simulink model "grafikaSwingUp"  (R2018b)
settings: Solver=ode4  StartTime=0.0  StopTime=1.85  FixedStep=1e-3  RelTol=1e-3
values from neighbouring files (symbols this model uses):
  dtheta0 = [dtheta0 , stbVc]    [mainSkript_provedeniSimulaceSwingUp.m]    (also in mainSkript_odhadKyvadlaZvlast.m = mean(dtheta(n_start-5:n_start+5)); mainSkript_pocitaniTVLQR_simplified.m = traj.dth_0)
  dtheta1 = [dtheta1 , stbVc]    [mainSkript_provedeniSimulaceSwingUp.m]    (also in mainSkript_pocitaniTVLQR_simplified.m = traj.dth_1)
  dtheta2 = [dtheta2 , stbVc]    [mainSkript_provedeniSimulaceSwingUp.m]    (also in mainSkript_pocitaniTVLQR_simplified.m = traj.dth_2)
  g = 9.81    [mainSkript_provedeniSimulaceSwingUp.m]    (also in mainSkript_rovniceSystemu.m; mainSkript_overeniRovnic.m; mainSkript_estimaceVozik.m; mainSkript_odhadKyvadlaZvlast.m)
  I_1 = params.I_1    [mainSkript_provedeniSimulaceSwingUp.m]    (also in mainSkript_rovniceSystemu.m; mainSkript_overeniRovnic.m; mainSkript_kyvadlaNajednouOdhad.m; mainSkript_simulaceLQG.m)
  I_2 = params.I_2    [mainSkript_provedeniSimulaceSwingUp.m]    (also in mainSkript_rovniceSystemu.m; mainSkript_overeniRovnic.m; mainSkript_kyvadlaNajednouOdhad.m; mainSkript_simulaceLQG.m)
  l_1 = params.l_1    [mainSkript_provedeniSimulaceSwingUp.m]    (also in mainSkript_rovniceSystemu.m; mainSkript_overeniRovnic.m; odhadovane_parametry.m = 0.134; mainSkript_kyvadlaNajednouOdhad.m)
  L_1 = params.L_1    [mainSkript_provedeniSimulaceSwingUp.m]    (also in mainSkript_rovniceSystemu.m; mainSkript_overeniRovnic.m; odhadovane_parametry.m = 0.228; mainSkript_kyvadlaNajednouOdhad.m)
  l_2 = params.l_2    [mainSkript_provedeniSimulaceSwingUp.m]    (also in mainSkript_rovniceSystemu.m; mainSkript_overeniRovnic.m; odhadovane_parametry.m = 0.112; mainSkript_kyvadlaNajednouOdhad.m)
  m = params.m_0    [mainSkript_estimaceVozik.m]    (also in mainSkript_odhadKyvadlaZvlast.m = params.m_2; mainSkript_modifikaceVozik.m = 1.437)
  m_0 = params.m_0    [mainSkript_provedeniSimulaceSwingUp.m]    (also in mainSkript_rovniceSystemu.m; mainSkript_overeniRovnic.m; mainSkript_simulaceLQG.m; mainSkript_LQGexperiment.m)
  m_1 = params.m_1    [mainSkript_provedeniSimulaceSwingUp.m]    (also in mainSkript_rovniceSystemu.m; mainSkript_overeniRovnic.m; mainSkript_kyvadlaNajednouOdhad.m; mainSkript_simulaceLQG.m)
  m_2 = params.m_2    [mainSkript_provedeniSimulaceSwingUp.m]    (also in mainSkript_rovniceSystemu.m; mainSkript_overeniRovnic.m; mainSkript_kyvadlaNajednouOdhad.m; mainSkript_simulaceLQG.m)
  N = N * Cref'    [mainSkript_simulaceLQG.m]    (also in mainSkript_tvorbaTrajektorii.m = 100; mainSkript_pocitaniTVLQR_simplified.m = floor( length(time) / krok ))
  theta0 = [theta0 , stbVc]    [mainSkript_provedeniSimulaceSwingUp.m]    (also in mainSkript_odhadKyvadlaZvlast.m = theta_cut(1); mainSkript_pocitaniTVLQR_simplified.m = traj.th_0)
  theta1 = [theta1 , stbVc]    [mainSkript_provedeniSimulaceSwingUp.m]    (also in mainSkript_kyvadlaNajednouOdhad.m = pend.theta1; mainSkript_pocitaniTVLQR_simplified.m = traj.th_1)
  theta2 = [theta2 , stbVc]    [mainSkript_provedeniSimulaceSwingUp.m]    (also in mainSkript_kyvadlaNajednouOdhad.m = pend.theta2; mainSkript_pocitaniTVLQR_simplified.m = traj.th_2)
undefined symbols (not defined in the file or in its folder): DiscIntNeverNeededParam, kg, rad, s
libraries: mblibv1 x14

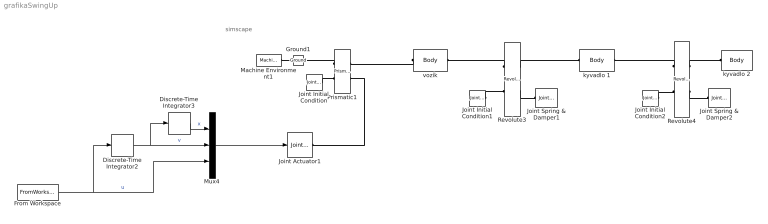
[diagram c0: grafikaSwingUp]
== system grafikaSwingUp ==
  note: simscape
  Discrete-Time Integrator2 : DiscreteIntegrator  SampleTime=1e-3  ICPrevOutput=DiscIntNeverNeededParam  ICPrevScaledInput=DiscIntNeverNeededParam
  Discrete-Time Integrator3 : DiscreteIntegrator  SampleTime=1e-3  ICPrevOutput=DiscIntNeverNeededParam  ICPrevScaledInput=DiscIntNeverNeededParam
  From Workspace : FromWorkspace  VariableName=u_str  SampleTime=0
  Ground1 : mblibv1/Bodies/Ground  UpdateFromCAD=off  LeftPortType=env  RightPortType=workingframe  PhysicalDomain=Mechanical  DialogClass=GroundBlock  CoordPosition=[0 0 0]  CoordPositionUnits=m  StateVectorMgrId=0  MachineId=[1 0]  ShowEnvPort=on  ParameterChecksum=[1834074738, 1660941931, 768696267, 1500060636]  TopologyChecksum=[1367285865, 302751694, 2522931292, 506890735]
  Joint Actuator1 : mblibv1/Sensors &  Actuators/Joint Actuator  UpdateFromCAD=off  PhysicalDomain=Mechanical  PortType=blob  ActuationStyle=Motion  AngleUnits=rad  ArcVelocityUnits=rad/s  ArcAccelerationUnits=rad/s^2  CoordPositionUnits=m  VelocityUnits=m/s  AccelerationUnits=m/s^2  ForceUnits=N  TorqueUnits=N*m  ActiveIO=on  Width=3  DialogClass=MechanicalActuatorBlock  Primitive=P1  ReferenceFrame=Absolute (World)
  Joint Initial Condition : mblibv1/Sensors &  Actuators/Joint Initial Condition  UpdateFromCAD=off  LeftPortType=blob  RightPortType=blob  PhysicalDomain=mechanical  DialogClass=InitialConditionBlock  InitialConditions=P1$true$theta0(1)$m$deg$dtheta0(1)$m/s$deg/s#P2$false$0$m$deg$0$m/s$deg/s#P3$false$0$m$deg$0$m/s$deg/s#R1$false$0$m$deg$0$m/s$deg/s#R2$false$0$m$deg$0$m/s$deg/s#R3$false$0$m$deg$0$m/s$deg/s#S$false$0$m$deg$0$m/s$deg/s  P1PIC=theta0(1)  P1VIC=dtheta0(1)  P2PIC=0  P2VIC=0  P3PIC=0  P3VIC=0  R1PIC=0  R1VIC=0  R2PIC=0  R2VIC=0  R3PIC=0  R3VIC=0  SPIC=0  SVIC=0
  Joint Initial Condition1 : mblibv1/Sensors &  Actuators/Joint Initial Condition  UpdateFromCAD=off  LeftPortType=blob  RightPortType=blob  PhysicalDomain=mechanical  DialogClass=InitialConditionBlock  InitialConditions=P1$false$th0i$m$deg$dth0i$m/s$deg/s#P2$false$0$m$deg$0$m/s$deg/s#P3$false$0$m$deg$0$m/s$deg/s#R1$true$theta1(1)$m$rad$dtheta1(1)$m/s$rad/s#R2$false$0$m$deg$0$m/s$deg/s#R3$false$0$m$deg$0$m/s$deg/s#S$false$0$m$deg$0$m/s$deg/s  P1PIC=0  P1VIC=0  P2PIC=0  P2VIC=0  P3PIC=0  P3VIC=0  R1PIC=theta1(1)  R1VIC=dtheta1(1)  R2PIC=0  R2VIC=0  R3PIC=0  R3VIC=0  SPIC=0  SVIC=0
  Joint Initial Condition2 : mblibv1/Sensors &  Actuators/Joint Initial Condition  UpdateFromCAD=off  LeftPortType=blob  RightPortType=blob  PhysicalDomain=mechanical  DialogClass=InitialConditionBlock  InitialConditions=P1$false$th0i$m$deg$dth0i$m/s$deg/s#P2$false$0$m$deg$0$m/s$deg/s#P3$false$0$m$deg$0$m/s$deg/s#R1$true$theta2(1) - theta1(1)$m$rad$dtheta2(1) - dtheta1(1)$m/s$rad/s#R2$false$0$m$deg$0$m/s$deg/s#R3$false$0$m$deg$0$m/s$deg/s#S$false$0$m$deg$0$m/s$deg/s  P1PIC=0  P1VIC=0  P2PIC=0  P2VIC=0  P3PIC=0  P3VIC=0  R1PIC=theta2(1) - theta1(1)  R1VIC=dtheta2(1) - dtheta1(1)  R2PIC=0  R2VIC=0  R3PIC=0  R3VIC=0  SPIC=0  SVIC=0
  Joint Spring & Damper1 : mblibv1/Force  Elements/Joint Spring & Damper  UpdateFromCAD=off  DialogClass=JointSpringDamper  JFEParameters=P1$false$0$b0$0$m$m/s$N$deg$deg/s$N*m#P2$false$0$0$0$m$m/s$N$deg$deg/s$N*m#P3$false$0$0$0$m$m/s$N$deg$deg/s$N*m#R1$true$0$b_1$0$m$m/s$N$rad$rad/s$N*m#R2$false$0$0$0$m$m/s$N$deg$deg/s$N*m#R3$false$0$0$0$m$m/s$N$deg$deg/s$N*m#S$false$0$0$0$m$m/s$N$deg$deg/s$N*m
  Joint Spring & Damper2 : mblibv1/Force  Elements/Joint Spring & Damper  UpdateFromCAD=off  DialogClass=JointSpringDamper  JFEParameters=P1$false$0$b0$0$m$m/s$N$deg$deg/s$N*m#P2$false$0$0$0$m$m/s$N$deg$deg/s$N*m#P3$false$0$0$0$m$m/s$N$deg$deg/s$N*m#R1$true$0$b_2$0$m$m/s$N$rad$rad/s$N*m#R2$false$0$0$0$m$m/s$N$deg$deg/s$N*m#R3$false$0$0$0$m$m/s$N$deg$deg/s$N*m#S$false$0$0$0$m$m/s$N$deg$deg/s$N*m
  Machine Environment1 : mblibv1/Bodies/Machine Environment  PortType=env  PhysicalDomain=Mechanical  DialogTemplateClass=MECH.MachineEnvironment  SyncWhenCopied=off  Gravity=[0 -g 0]  GravityUnits=m/s^2  GravityAsSignal=off  Dimensionality=Auto-detect  AnalysisType=Forward dynamics  LinearAssemblyTolerance=1e-3  LinearAssemblyToleranceUnits=m  AngularAssemblyTolerance=1e-3  AngularAssemblyToleranceUnits=rad  ConstraintSolverType=Stabilizing  ConstraintRelTolerance=1e-4  ConstraintAbsTolerance=1e-4  UseRobustSingularityHandling=off  RedundancyAnalysisToleranceType=Automatically select tolerance  RedundancyAnalysisTolerance=1e-14  StatePerturbationType=Fixed  PerturbationSize=1e-5  VisualizeMachine=on  BodyVisualizationType=Use model default body geometries  BodyColorSelMode=Use model default  DefaultBodyColor=[1 0 0]
  Mux4 : Mux  Inputs=3
  Prismatic1 : mblibv1/Joints/Prismatic  LConnTagsString=__newl0|SA1  RConnTagsString=__newr0|SA1  UpdateFromCAD=off  NumSAPorts=2  CutJoint=off  MarkAsCut=off  Primitives=prismatic  PrimitiveProps=P1$World$[-1 0 0]$prismatic  DialogClass=JointBlock  P1Axis=[-1 0 0]
  Revolute3 : mblibv1/Joints/Revolute  LConnTagsString=__newl0|SA1  RConnTagsString=__newr0|SA1  UpdateFromCAD=off  NumSAPorts=2  CutJoint=off  MarkAsCut=off  Primitives=prismatic  PrimitiveProps=R1$World$[0 0 1]$revolute  DialogClass=JointBlock  R1Axis=[0 0 1]
  Revolute4 : mblibv1/Joints/Revolute  LConnTagsString=__newl0|SA1  RConnTagsString=__newr0|SA1  UpdateFromCAD=off  NumSAPorts=2  CutJoint=off  MarkAsCut=off  Primitives=prismatic  PrimitiveProps=R1$Base$[0 0 1]$revolute  DialogClass=JointBlock  R1Axis=[0 0 1]
  kyvadlo 1 : mblibv1/Bodies/Body  LConnTagsString=CS1  RConnTagsString=CS2  UpdateFromCAD=off  DialogClass=MechanicalBodyBlock  Mass=m_1  MassUnits=kg  InertiaUnits=kg*m^2  Inertia=eye(3)*I_1  Shape=Cylinder  ShapeDims=[1 1]  ShapeUnits=m  ShapeUse=false  Density=1  DensityUnits=kg/m^3  DensityUse=false  GraphicsMode=MACHINE_DEFAULT  BodyColorSelMode=COLORPALETTE  BodyColor=[0 0 0]  AttachedToCS=CG  CG=Left$CG$[0 l_1 0]$CS1$CS1$m$[0 0 0]$Euler X-Y-Z$deg$WORLD$false$none  WorkingFrames=Left$CS1$[0 0 0]$Adjoining$Adjoining$m$[0 0 0]$Euler X-Y-Z$deg$WORLD$true$none#Right$CS2$[0 L_1 0]$CS1$CS1$m$[0 0 0]$Euler X-Y-Z$deg$WORLD$true$none  CGPos=[0 l_1 0]  CGRot=[0 0 0]  CS0Pos=[]  CS0Rot=[]  CS1Pos=[0 0 0]  CS1Rot=[0 0 0]  CS2Pos=[0 L_1 0]  CS2Rot=[0 0 0]  CS3Pos=[]  CS3Rot=[]  CS4Pos=[]  CS4Rot=[]  CS5Pos=[]  CS5Rot=[]  CS6Pos=[]  CS6Rot=[]  CS7Pos=[]  CS7Rot=[]  CS8Pos=[]  CS8Rot=[]  CS9Pos=[]  CS9Rot=[]  CS10Pos=[]  CS10Rot=[]  CS11Pos=[]  CS11Rot=[]  CS12Pos=[]  CS12Rot=[]  CS13Pos=[]  CS13Rot=[]  CS14Pos=[]  CS14Rot=[]  CS15Pos=[]  CS15Rot=[]  CS16Pos=[]  CS16Rot=[]  CS17Pos=[]  CS17Rot=[]  CS18Pos=[]  CS18Rot=[]  CS19Pos=[]  CS19Rot=[]  CS20Pos=[]  CS20Rot=[]
  kyvadlo 2 : mblibv1/Bodies/Body  LConnTagsString=CS1  RConnTagsString=CS2  UpdateFromCAD=off  DialogClass=MechanicalBodyBlock  Mass=m_2  MassUnits=kg  InertiaUnits=kg*m^2  Inertia=eye(3)*I_2  Shape=Cylinder  ShapeDims=[1 1]  ShapeUnits=m  ShapeUse=false  Density=1  DensityUnits=kg/m^3  DensityUse=false  GraphicsMode=MACHINE_DEFAULT  BodyColorSelMode=COLORPALETTE  BodyColor=[0 0 0]  AttachedToCS=CG  CG=Left$CG$[0 l_2 0]$CS1$CS1$m$[0 0 0]$Euler X-Y-Z$deg$WORLD$false$none  WorkingFrames=Left$CS1$[0 0 0]$Adjoining$Adjoining$m$[0 0 0]$Euler X-Y-Z$deg$WORLD$true$none#Right$CS2$[0 2*l_2 0]$CS1$CS1$m$[0 0 0]$Euler X-Y-Z$deg$WORLD$true$none  CGPos=[0 l_2 0]  CGRot=[0 0 0]  CS0Pos=[]  CS0Rot=[]  CS1Pos=[0 0 0]  CS1Rot=[0 0 0]  CS2Pos=[0 2*l_2 0]  CS2Rot=[0 0 0]  CS3Pos=[]  CS3Rot=[]  CS4Pos=[]  CS4Rot=[]  CS5Pos=[]  CS5Rot=[]  CS6Pos=[]  CS6Rot=[]  CS7Pos=[]  CS7Rot=[]  CS8Pos=[]  CS8Rot=[]  CS9Pos=[]  CS9Rot=[]  CS10Pos=[]  CS10Rot=[]  CS11Pos=[]  CS11Rot=[]  CS12Pos=[]  CS12Rot=[]  CS13Pos=[]  CS13Rot=[]  CS14Pos=[]  CS14Rot=[]  CS15Pos=[]  CS15Rot=[]  CS16Pos=[]  CS16Rot=[]  CS17Pos=[]  CS17Rot=[]  CS18Pos=[]  CS18Rot=[]  CS19Pos=[]  CS19Rot=[]  CS20Pos=[]  CS20Rot=[]
  vozík : mblibv1/Bodies/Body  LConnTagsString=CS1  RConnTagsString=CS2  UpdateFromCAD=off  DialogClass=MechanicalBodyBlock  Mass=m_0  MassUnits=kg  InertiaUnits=kg*m^2  Inertia=zeros(3)  Shape=Cylinder  ShapeDims=[1 1]  ShapeUnits=m  ShapeUse=false  Density=1  DensityUnits=kg/m^3  DensityUse=false  GraphicsMode=MACHINE_DEFAULT  BodyColorSelMode=COLORPALETTE  BodyColor=[0 0 0]  AttachedToCS=CG  CG=Left$CG$[0 0 0]$WORLD$WORLD$m$[0 0 0]$Euler X-Y-Z$deg$WORLD$false$none  WorkingFrames=Left$CS1$[0 0 0]$CG$CG$m$[0 0 0]$Euler X-Y-Z$deg$WORLD$true$none#Right$CS2$[0 0 0]$CG$CG$m$[0 0 0]$Euler X-Y-Z$deg$WORLD$true$none  CGPos=[0 0 0]  CGRot=[0 0 0]  CS0Pos=[]  CS0Rot=[]  CS1Pos=[0 0 0]  CS1Rot=[0 0 0]  CS2Pos=[0 0 0]  CS2Rot=[0 0 0]  CS3Pos=[]  CS3Rot=[]  CS4Pos=[]  CS4Rot=[]  CS5Pos=[]  CS5Rot=[]  CS6Pos=[]  CS6Rot=[]  CS7Pos=[]  CS7Rot=[]  CS8Pos=[]  CS8Rot=[]  CS9Pos=[]  CS9Rot=[]  CS10Pos=[]  CS10Rot=[]  CS11Pos=[]  CS11Rot=[]  CS12Pos=[]  CS12Rot=[]  CS13Pos=[]  CS13Rot=[]  CS14Pos=[]  CS14Rot=[]  CS15Pos=[]  CS15Rot=[]  CS16Pos=[]  CS16Rot=[]  CS17Pos=[]  CS17Rot=[]  CS18Pos=[]  CS18Rot=[]  CS19Pos=[]  CS19Rot=[]  CS20Pos=[]  CS20Rot=[]
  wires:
  From Workspace/1 -> Mux4/3, Discrete-Time Integrator2/1  "u"
  Discrete-Time Integrator2/1 -> Mux4/2, Discrete-Time Integrator3/1  "v"
  Discrete-Time Integrator3/1 -> Mux4/1  "x"
  Mux4/1 -> Joint Actuator1/1
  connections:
  Joint Initial Condition2/RConn1 -- Revolute4/LConn2
  vozík/LConn1 -- Prismatic1/RConn1
  Joint Initial Condition1/RConn1 -- Revolute3/LConn2
  Prismatic1/LConn1 -- Ground1/RConn1
  Revolute3/RConn1 -- kyvadlo 1/LConn1
  Revolute4/RConn1 -- kyvadlo 2/LConn1
  Revolute3/LConn1 -- vozík/RConn1
  Revolute4/LConn1 -- kyvadlo 1/RConn1
  Revolute3/RConn2 -- Joint Spring & Damper1/LConn1
  Machine Environment1/RConn1 -- Ground1/LConn1
  Revolute4/RConn2 -- Joint Spring & Damper2/LConn1
  Joint Initial Condition/RConn1 -- Prismatic1/LConn2
  Joint Actuator1/RConn1 -- Prismatic1/RConn2
